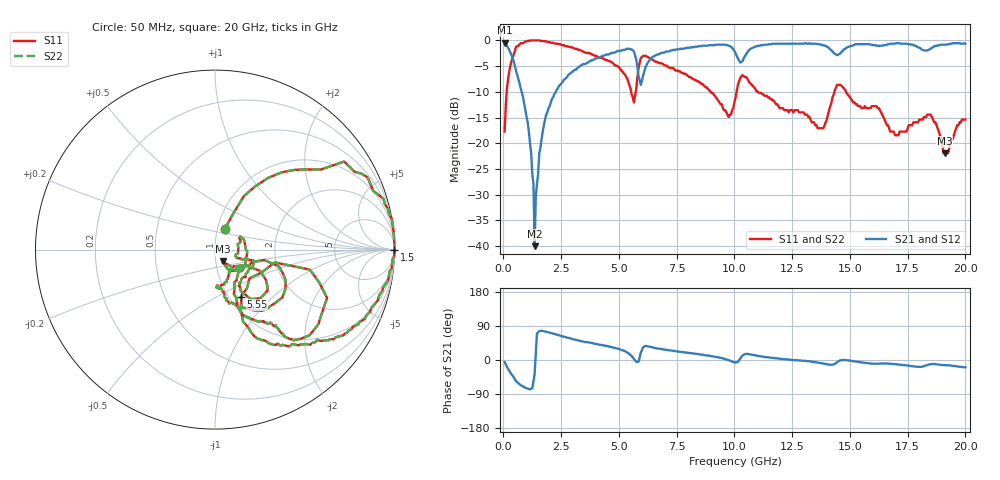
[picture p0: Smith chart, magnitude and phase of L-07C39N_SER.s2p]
#	mhz	s	ma	r	50
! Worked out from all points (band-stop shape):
!   400 points, 50 MHz to 20 GHz, reference 50 ohm
!   highest |S21| = -0.45 dB at 50 MHz (marker M1); lowest = -40.0 dB at 1.35 GHz (marker M2)
!   |S21| within 3 dB of the highest: 6.406 GHz to 10.15 GHz (3.74 GHz wide, 45.2 % of centre); 10.4 GHz to end of sweep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
!   lowest |S11| = -21.9 dB at 19.1 GHz (marker M3), VSWR 1.17, Z = 54.3 - j7.18 ohm
!   |S11| at or under -10 dB: 8.969 GHz to 10.1 GHz (1.127 GHz wide, 11.8 % of centre); 11.02 GHz to 14.33 GHz (3.309 GHz wide, 26.1 % of centre); 14.83 GHz to end of sweep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
!   |S22| runs from -21.9 to 0.0 dB; largest |S21 - S12| = 0
!   S11 on the Smith chart (normalised r, x): 50 MHz: 1.09, +0.26; 1.5 GHz: open; 5.55 GHz: 1.13, -0.66; 20 GHz: 1.28, -0.27
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50  0.13 64.7  0.95 -5.5  0.95 -5.5  0.13 64.7
300  0.57 49.1  0.76 -33.2  0.76 -33.2  0.57 49.1
1050  0.99 13.2  0.16 -75.7  0.16 -75.7  0.99 13.2
1300  1 5.6  0.04 -55.6  0.04 -55.6  1 5.6
1350  1 3.7  0.01 -36.8  0.01 -36.8  1 3.7
1400  1 2.6  0.03 16.4  0.03 16.4  1 2.6
1500  1 -0.2  0.05 73.0  0.05 73.0  1 -0.2
2100  0.95 -16.3  0.27 70.5  0.27 70.5  0.95 -16.3
3400  0.79 -39.9  0.58 49.3  0.58 49.3  0.79 -39.9
5550  0.3 -61.3  0.82 10.8  0.82 10.8  0.3 -61.3
5950  0.68 -23.3  0.37 19.7  0.37 19.7  0.68 -23.3
6700  0.61 -51.2  0.73 30.1  0.73 30.1  0.61 -51.2
9750  0.18 -43.4  0.89 -0.4  0.89 -0.4  0.18 -43.4
10050  0.28 -11.9  0.75 -6.6  0.75 -6.6  0.28 -11.9
10550  0.43 -52.4  0.76 16.3  0.76 16.3  0.43 -52.4
13350  0.16 -61.4  0.93 -4.4  0.93 -4.4  0.16 -61.4
13850  0.14 -41.1  0.9 -9.4  0.9 -9.4  0.14 -41.1
14600  0.37 -46.7  0.76 -0.9  0.76 -0.9  0.37 -46.7
16700  0.14 -20.0  0.92 -9.7  0.92 -9.7  0.14 -20.0
18500  0.19 -38.1  0.83 -11.0  0.83 -11.0  0.19 -38.1
19100  0.08 -55.2  0.91 -13.5  0.91 -13.5  0.08 -55.2
20000  0.17 -36.8  0.93 -19.3  0.93 -19.3  0.17 -36.8
